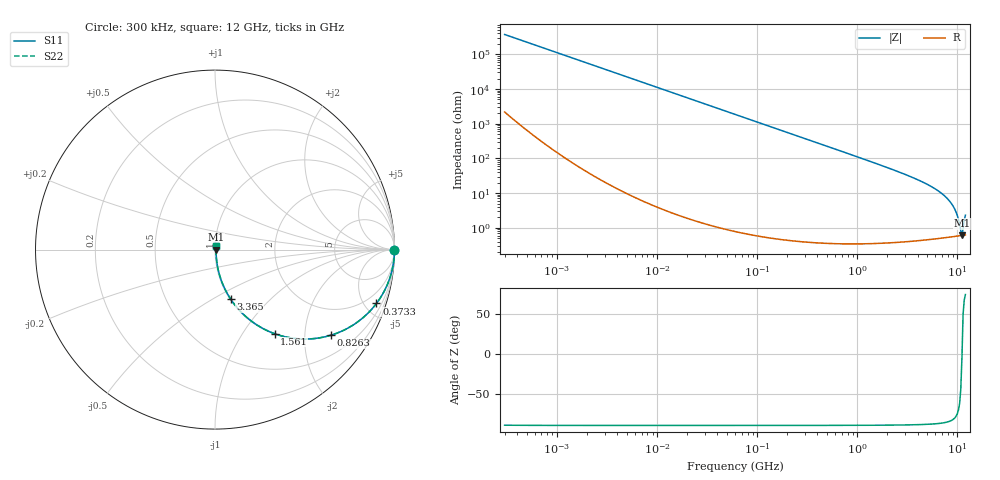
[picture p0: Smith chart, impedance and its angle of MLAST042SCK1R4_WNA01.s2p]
! MLAST042SCK1R4_WNA01  S-PARAMETER MODEL  ( General Type )
! Model Generated by TAIYO YUDEN Corporation (http://www.ty-top.com)
! Version 1.0
! TAIYO YUDEN Control No. 150820
! Copyright(c) 2015 TAIYO YUDEN CO.,LTD. All Rights Reserved.
! Product Description (link to TY-COMPAS)
! https://ds.yuden.co.jp/TYCOMPAS/or/detail?pn=MLAST042SCK1R4AWNA01&u=M
! Products Name : Multilayer Ceramic Capacitors
! Characteristics :
!  Capacitance : 1.4 pF , Rated Voltage : 25V , TCC : CK / C0K
!  Case Size : 0.4 x 0.2 / 0.016 x 0.008 [mm/inch] , Thickness : 0.2 / 0.008 [mm/inch]
!  (Conditions: Temperature = 25 degC , DC Bias Current/Voltage = 0A / 0V)
! External Node Assignments :
!  1  o---| |---o  2
! GND o---------o GND
! Frequency Range : 0.3MHz  -  12000MHz  [ 401 STEP ]
# MHz S RI R 50
! Freq[MHz].  S11 Real  S11 Imag  S21 Real  S21 Imag  S12 Real  S12 Imag  S22 Real  S22 Imag
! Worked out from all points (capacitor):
!   401 points, 300 kHz to 12 GHz, reference 50 ohm
!   read as one part in series: C = 1.42 pF near 316.3 kHz
!   lowest |Z| = 605 mohm at 11.08 GHz (marker M1)
!   series resonance near 11.1 GHz, so ESL is about 140 pH
!   S11 on the Smith chart (normalised r, x): 300 kHz: open; 373.3 MHz: 1.01, -5.99; 826.3 MHz: 1.01, -2.69; 1.561 GHz: 1.01, -1.41; 3.365 GHz: 1.01, -0.60; 12 GHz: 1.01, +0.04
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0.3  1 -0.000268  1.64e-06 0.000268  1.64e-06 0.000268  1 -0.000268
1.769972  1 -0.00158  3.76e-06 0.00158  3.76e-06 0.00158  1 -0.00158
10.44266  0.9999 -0.00933  9.03e-05 0.00933  9.03e-05 0.00933  0.9999 -0.00933
60  0.9971 -0.0535  0.00289 0.0535  0.00289 0.0535  0.9971 -0.0535
155.7172  0.9809 -0.1365  0.0191 0.1365  0.0191 0.1365  0.9809 -0.1365
353.9943  0.9086 -0.2876  0.0914 0.2876  0.0914 0.2876  0.9086 -0.2876
373.2558  0.8994 -0.3002  0.1006 0.3002  0.1006 0.3002  0.8994 -0.3002
555.3718  0.8012 -0.3982  0.1988 0.3982  0.1988 0.3982  0.8012 -0.3982
826.3444  0.6443 -0.4775  0.3557 0.4775  0.3557 0.4775  0.6443 -0.4775
1560.575  0.3315 -0.4683  0.6685 0.4683  0.6685 0.4683  0.3315 -0.4683
2088.533  0.2125 -0.4056  0.7875 0.4056  0.7875 0.4056  0.2125 -0.4056
3364.605  0.0867 -0.2748  0.9133 0.2748  0.9133 0.2748  0.0867 -0.2748
5565.855  0.0265 -0.146  0.9735 0.146  0.9735 0.146  0.0265 -0.146
7648.807  0.011 -0.0758  0.989 0.0758  0.989 0.0758  0.011 -0.0758
8503.825  0.00831 -0.0538  0.9917 0.0538  0.9917 0.0538  0.00831 -0.0538
9207.246  0.00699 -0.0376  0.993 0.0376  0.993 0.0376  0.00699 -0.0376
9968.853  0.00621 -0.0217  0.9938 0.0217  0.9938 0.0217  0.00621 -0.0217
10511.28  0.00599 -0.0111  0.994 0.0111  0.994 0.0111  0.00599 -0.0111
10793.46  0.00596 -0.00578  0.994 0.00578  0.994 0.00578  0.00596 -0.00578
11083.22  0.006 -0.000527  0.994 0.000527  0.994 0.000527  0.006 -0.000527
11380.75  0.00611 0.00711  0.9939 -0.00711  0.9939 -0.00711  0.00611 0.00711
12000  0.00668 0.0219  0.9933 -0.0219  0.9933 -0.0219  0.00668 0.0219
